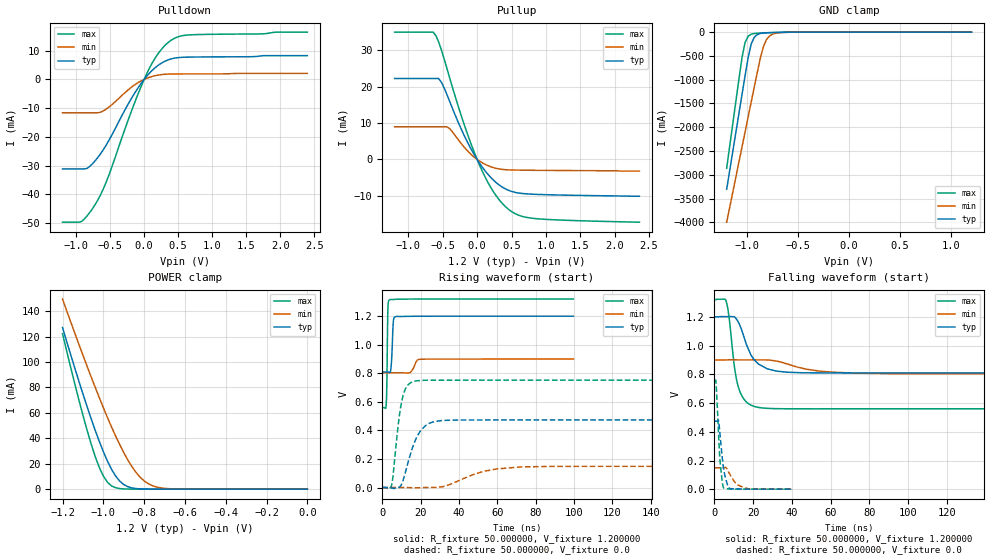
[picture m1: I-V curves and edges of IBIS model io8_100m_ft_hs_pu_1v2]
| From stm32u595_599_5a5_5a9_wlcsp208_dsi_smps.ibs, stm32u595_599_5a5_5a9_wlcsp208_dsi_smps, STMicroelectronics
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|   Model io8_100m_ft_hs_pu_1v2
[Model]  io8_100m_ft_hs_pu_1v2
Model_type I/O
Polarity   Non-Inverting
Enable   Active-Low
Vinl =   0.360000V
Vinh =   0.840000V
Vmeas =  0.600000V
Cref =   50.000000pF
Rref =   100.000000M
Vref =   0.0V
C_comp   2.947800pF   2.877700pF   2.996100pF
[Temperature Range]   25.000000   0.140000k   -40.000000
[Pullup Reference]   1.200000V   0.900000V   1.320000V
[Pulldown Reference]   0.0V   0.0V   0.0V
[POWER Clamp Reference]   1.200000V   0.900000V   1.320000V
[GND Clamp Reference]   0.0V   0.0V   0.0V
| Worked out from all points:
|   slope of the pulldown table from 0 to 0.18 V, typ, clamps not added: 40.7 ohm
|   slope of the pullup table from 0 to 0.18 V, typ, clamps not added: 39.5 ohm
|   GND clamp passes 1 mA (typ) near -0.51 V on its own axis
|   POWER clamp passes 1 mA (typ) near -0.86 V on its own axis
|   rising waveform, R_fixture 50.000000, V_fixture 1.200000: 20-80 % time 753ps typ, 2.05ns min, 443ps max; typ from 0.809 V to 1.2 V
|   rising waveform, R_fixture 50.000000, V_fixture 0.0: 20-80 % time 7.29ns typ, 18.3ns min, 3.99ns max; typ from 0.001 V to 0.474 V
|   falling waveform, R_fixture 50.000000, V_fixture 1.200000: 20-80 % time 7.87ns typ, 18.4ns min, 4.53ns max; typ from 1.2 V to 0.809 V
|   falling waveform, R_fixture 50.000000, V_fixture 0.0: 20-80 % time 2.51ns typ, 4.78ns min, 1.85ns max; typ from 0.474 V to 0.001 V
[Pulldown]
|Voltage   I(typ)   I(min)   I(max)
-1.2V     -31.16mA   -11.61mA   -49.71mA
-920mV    -31.16mA   -11.61mA   -49.49mA
-840mV    -31mA      -11.61mA   -47.54mA
-720mV    -28.32mA   -11.61mA   -43.58mA
-560mV    -22.95mA   -10.37mA   -35.89mA
-200mV    -7.146mA   -2.964mA   -11.89mA
0V        0A         0A         0A
160mV     4.047mA    1.298mA    7.361mA
360mV     6.869mA    1.87mA     13mA
480mV     7.543mA    1.91mA     14.69mA
640mV     7.765mA    1.923mA    15.46mA
2.4V      8.291mA    2.091mA    16.49mA
[Pullup]
|Voltage   I(typ)   I(min)   I(max)
-1.2V     22.25mA    8.963mA    34.99mA
-640mV    22.25mA    8.963mA    34.99mA
-600mV    22.25mA    8.963mA    34.03mA
-520mV    21.23mA    8.963mA    30.12mA
-400mV    15.99mA    8.489mA    22.45mA
-200mV    7.069mA    3.642mA    10.26mA
0V        550fA      209pA      10fA
240mV     -5.73mA    -2.256mA   -8.953mA
480mV     -8.639mA   -2.877mA   -14.04mA
640mV     -9.31mA    -2.942mA   -15.55mA
880mV     -9.601mA   -2.986mA   -16.29mA
2.36V     -10.1mA    -3.2mA     -17.23mA
[GND_clamp]
|Voltage   I(typ)   I(min)   I(max)
-1.2V     -3.305A    -3.998A    -2.862A
-1.05V    -1.316A    -2.418A    -539.3mA
-1.02V    -921mA     -2.103A    -218.8mA
-990mV    -539.5mA   -1.788A    -87.43mA
-960mV    -252.1mA   -1.474A    -44.36mA
-930mV    -110.5mA   -1.16A     -30.32mA
-870mV    -28.03mA   -549.1mA   -21.09mA
-840mV    -18.43mA   -305.6mA   -18.27mA
-810mV    -13.9mA    -159.7mA   -15.73mA
-780mV    -11.23mA   -82.35mA   -13.37mA
-600mV    -2.976mA   -4.272mA   -3.058mA
1.2V      0A         14.74nA    0A
[POWER_clamp]
|Voltage   I(typ)   I(min)   I(max)
-1.2V     127mA      149.4mA    122.2mA
-1.12V    84.98mA    114mA      70.29mA
-1.06V    55.52mA    88.42mA    35.69mA
-1.02V    37.64mA    72.04mA    17.19mA
-1V       29.52mA    64.13mA    10.33mA
-960mV    15.7mA     48.99mA    2.596mA
-900mV    3.636mA    28.77mA    207.8uA
-840mV    502.9uA    13.24mA    43.4uA
-800mV    129uA      6.535mA    43.4uA
-740mV    25.52uA    1.726mA    43.4uA
-620mV    25.17uA    82.33uA    35.63uA
0V        0A         17.33nA    0A
[Ramp]
| variable   typ   min   max
dV/dt_r  0.28390/7.27930n   89.02186m/18.31659n 0.45096/3.97961n
dV/dt_f  0.23429/7.85372n   57.82800m/18.40475n 0.45608/4.52306n
R_load = 50.000000
[Rising Waveform]
R_fixture= 50.000000
V_fixture= 1.200000
V_fixture_min= 0.900000
V_fixture_max= 1.320000
|time   V(typ)   V(min)   V(max)
0s        809.5mV    803.6mV    559.9mV
2.002ns   809.5mV    803.6mV    576.1mV
2.402ns   809.5mV    803.6mV    767.5mV
2.803ns   809.4mV    803.6mV    1.212V
3.804ns   805.4mV    803.6mV    1.315V
4.605ns   852.8mV    803.6mV    1.317V
5.806ns   1.173V     803.6mV    1.317V
6.807ns   1.196V     803.6mV    1.318V
19.62ns   1.2V       898.1mV    1.32V
99.7ns    1.2V       900mV      1.32V
[Rising Waveform]
R_fixture= 50.000000
V_fixture= 0.0
V_fixture_min= 0.0
V_fixture_max= 0.0
|time   V(typ)   V(min)   V(max)
0s        593.5uV    601.1uV    547.1uV
4.805ns   -1.842mV   600.9uV    14.58mV
8.408ns   1.217mV    599.9uV    452.5mV
10.21ns   28.03mV    601.9uV    611mV
12.61ns   137.3mV    646.7uV    705.5mV
17.42ns   338.1mV    -865.8uV   746.6mV
22.82ns   437.3mV    813.1uV    751.7mV
34.23ns   471.6mV    17.23mV    752mV
72.67ns   473.7mV    145.1mV    752.1mV
299.1ns   473.8mV    149mV      752.1mV
[Falling Waveform]
R_fixture= 50.000000
V_fixture= 1.200000
V_fixture_min= 0.900000
V_fixture_max= 1.320000
|time   V(typ)   V(min)   V(max)
0s        1.2V       900mV      1.32V
6.006ns   1.201V     900.1mV    1.311V
7.608ns   1.202V     900.6mV    1.191V
10.41ns   1.2V       900.6mV    844.2mV
12.01ns   1.171V     900.5mV    727.6mV
15.62ns   1.044V     900.4mV    620.3mV
20.82ns   897.1mV    900.5mV    575.5mV
27.63ns   836.7mV    899.5mV    563mV
44.84ns   810.7mV    843.6mV    559.9mV
199.4ns   809.5mV    803.6mV    559.9mV
[Falling Waveform]
R_fixture= 50.000000
V_fixture= 0.0
V_fixture_min= 0.0
V_fixture_max= 0.0
|time   V(typ)   V(min)   V(max)
0s        473.8mV    149mV      752.1mV
800.8ps   473.8mV    149mV      743.8mV
2.162ns   474.3mV    149mV      372mV
2.963ns   369.7mV    149mV      185.3mV
4.565ns   159.2mV    149mV      13.23mV
6.567ns   37.58mV    138.7mV    3.411mV
7.928ns   4.753mV    104.2mV    1.955mV
11.61ns   2.225mV    34.73mV    921.5uV
17.38ns   1.027mV    3.652mV    632.8uV
39.88ns   593.5uV    601.1uV    547.1uV
